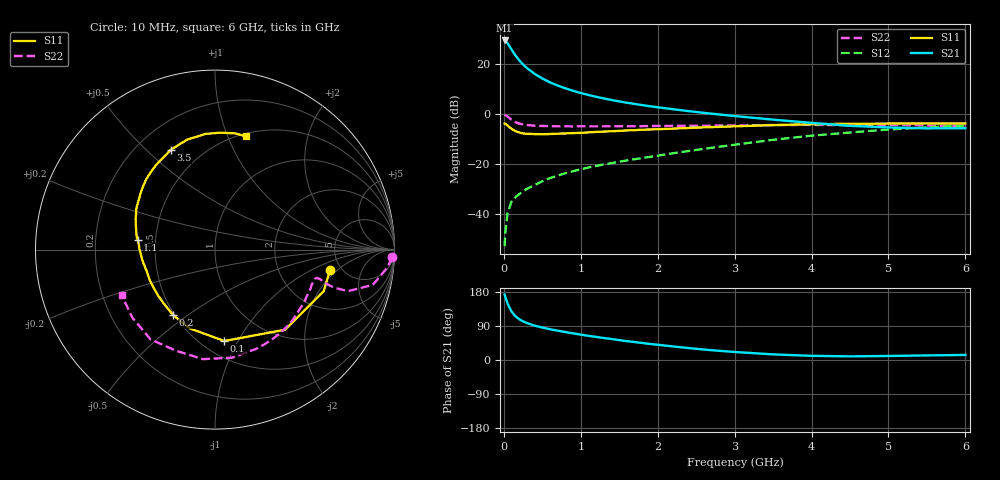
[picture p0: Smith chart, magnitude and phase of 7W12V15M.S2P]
! Infineon Technologies  Discrete & RF Semiconductors
! BFS17W
! Si NPN RF Bipolar Junction Transistor in SOT323
! VCE = 12 V  IC = 15 mA
! Common Emitter S-Parameters:  August  1999
# GHz  S  MA  R  50
!  f  S11  S21  S12  S22
! GHz  MAG  ANG  MAG  ANG  MAG  ANG  MAG  ANG
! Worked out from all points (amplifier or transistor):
!   36 points, 10 MHz to 6 GHz, reference 50 ohm
!   highest |S21| = 29.5 dB at 10 MHz (marker M1)
!   |S21| within 3 dB of that: start of sweep to 87.13 MHz
!   unconditionally stable (mu >= 1): 376.3 MHz to 2.03 GHz; 5.824 GHz to end of sweep
!   at 250 MHz: K = 0.86, MSG = 25.4 dB, |S12| = -30.9 dB
!   at 1.4 GHz: K = 1.14, MAG = 10.4 dB, |S12| = -19.6 dB
!   at 6 GHz: K = 1.01, MAG = -1.3 dB, |S12| = -4.5 dB
!   S11 on the Smith chart (normalised r, x): 10 MHz: 4.03, -1.62; 100 MHz: 0.64, -0.88; 200 MHz: 0.49, -0.44; 1.1 GHz: 0.40, +0.05; 3.5 GHz: 0.34, +0.60; 6 GHz: 0.53, +1.17
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0.01  0.6504 -10.3  30.02 172.9  0.0023 79.6  0.987 -2.5
0.02  0.6486 -21.0  29.47 166.0  0.0044 80.6  0.9669 -5.8
0.05  0.5929 -48.8  26.16 148.3  0.0108 69.8  0.901 -12.6
0.1  0.5118 -84.2  19.77 128.1  0.018 61.4  0.7755 -17.4
0.15  0.4611 -107.7  15.12 115.5  0.0219 58.4  0.6957 -17.7
0.2  0.4334 -122.6  12.06 107.7  0.0254 59.8  0.6519 -17.1
0.25  0.4145 -133.6  9.924 101.9  0.0285 59.6  0.6253 -16.3
0.3  0.4069 -142.1  8.415 97.6  0.0323 61.8  0.6108 -15.8
0.4  0.4021 -154.0  6.441 90.7  0.0386 63.6  0.5919 -15.5
0.5  0.3991 -161.6  5.203 85.6  0.0458 66.0  0.5844 -15.8
0.6  0.4033 -167.4  4.353 81.2  0.0529 68.0  0.5792 -16.5
0.7  0.4097 -172.3  3.761 77.3  0.0595 68.4  0.5762 -17.7
0.9  0.4213 179.6  2.95 70.3  0.0727 69.9  0.5728 -20.5
1.1  0.4347 172.6  2.435 63.8  0.0864 70.7  0.5739 -23.9
1.3  0.4511 166.4  2.076 58.0  0.0996 71.4  0.5736 -27.8
1.6  0.4759 158.4  1.702 49.8  0.1193 72.7  0.5764 -33.8
2.2  0.5172 143.7  1.263 35.7  0.1662 75.0  0.5873 -47.5
2.8  0.5611 129.5  0.992 24.2  0.2244 74.3  0.5953 -62.5
3.5  0.6083 113.9  0.782 14.8  0.3089 70.4  0.6098 -81.0
4.5  0.6467 94.7  0.588 9.6  0.4323 58.9  0.6036 -111.3
5.5  0.6573 80.3  0.523 12.1  0.5485 45.7  0.5962 -140.7
6  0.6546 74.7  0.527 13.4  0.5957 38.9  0.5789 -154.0
